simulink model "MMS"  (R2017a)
settings: Solver=VariableStepAuto  StartTime=0.0  StopTime=10.0  RelTol=1e-3
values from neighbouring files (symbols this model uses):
  d = 5    [MMS_init.m]
  f = 1    [MMS_init.m]
  k = 2    [MMS_init.m]
  m = 1    [MMS_init.m]
  p0 = 0    [MMS_init.m]

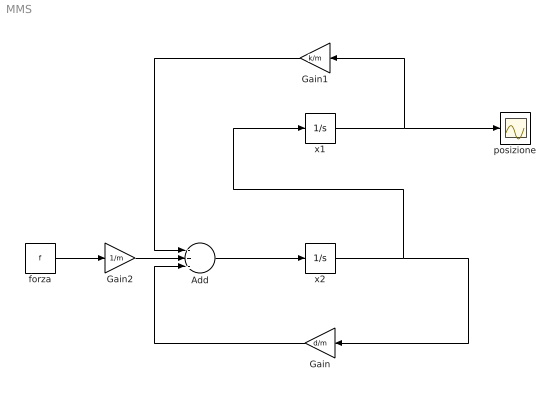
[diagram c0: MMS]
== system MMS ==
  Add : Sum  Inputs=-+-
  Gain : Gain  Gain=d/m
  Gain1 : Gain  Gain=k/m
  Gain2 : Gain  Gain=1/m
  forza : Constant  Value=f
  posizione : Scope
  x1 : Integrator  InitialCondition=p0
  x2 : Integrator
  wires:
  Add/1 -> x2/1
  Gain/1 -> Add/3
  x2/1 -> x1/1, Gain/1
  x1/1 -> Gain1/1, posizione/1
  Gain1/1 -> Add/1
  forza/1 -> Gain2/1
  Gain2/1 -> Add/2
